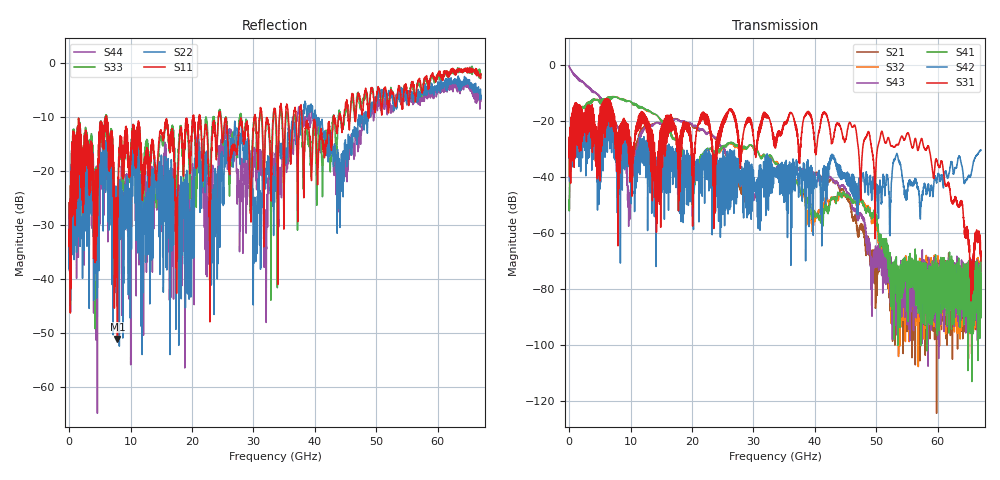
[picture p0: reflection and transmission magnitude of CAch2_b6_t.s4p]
!Agilent Technologies,N5247A,US51170199,A.09.90.13
!Agilent N5247A: A.09.90.13
!Date: Tuesday, October 23, 2018 12:56:16
!Correction: S11(Full 4 Port(1,2,3,4))
!S12(Full 4 Port(1,2,3,4))
!S13(Full 4 Port(1,2,3,4))
!S14(Full 4 Port(1,2,3,4))
!S21(Full 4 Port(1,2,3,4))
!S22(Full 4 Port(1,2,3,4))
!S23(Full 4 Port(1,2,3,4))
!S24(Full 4 Port(1,2,3,4))
!S31(Full 4 Port(1,2,3,4))
!S32(Full 4 Port(1,2,3,4))
!S33(Full 4 Port(1,2,3,4))
!S34(Full 4 Port(1,2,3,4))
!S41(Full 4 Port(1,2,3,4))
!S42(Full 4 Port(1,2,3,4))
!S43(Full 4 Port(1,2,3,4))
!S44(Full 4 Port(1,2,3,4))
!S4P File: Measurements: <S11,S12,S13,S14>,
!<S21,S22,S23,S24>,
!<S31,S32,S33,S34>,
!<S41,S42,S43,S44>:
# Hz S  dB  R 50
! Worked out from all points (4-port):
!   6701 points, 10 MHz to 67 GHz, reference 50 ohm
!   strongest paths, dB at 10 MHz, 16.76 GHz, 33.51 GHz, 50.25 GHz, 67 GHz:
!     S31: -33.0, -22.9, -27.3, -29.1, -70.0
!     S42: -33.4, -33.4, -36.8, -50.6, -30.5
!     S41: -48.3, -25.6, -35.4, -57.9, -68.5
!     S43: -0.5, -19.7, -37.8, -66.1, -68.7
!     S32: -48.4, -25.3, -35.1, -59.1, -70.9
!     S21: -0.5, -19.5, -37.4, -69.5, -80.2
!   lowest |S11| = -51.0 dB at 7.869 GHz (marker M1), VSWR 1.01, Z = 50.3 + j0.0174 ohm
!   |S11| at or under -10 dB: start of sweep to 5.977 GHz; 6.104 GHz to 20.16 GHz (14.05 GHz wide, 107 % of centre); 24.68 GHz to 30.15 GHz (5.474 GHz wide, 20 % of centre)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
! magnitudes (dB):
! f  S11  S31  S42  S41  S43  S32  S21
! 10 MHz  -25.9  -33.0  -33.4  -48.3  -0.5  -48.4  -0.5
! 7.869 GHz  -51.0  -30.2  -38.4  -11.7  -22.2  -11.6  -22.0
! 9.839 GHz  -20.3  -30.3  -34.6  -12.9  -49.5  -13.0  -34.1
! 19.61 GHz  -17.2  -25.6  -35.6  -44.0  -20.6  -41.7  -20.8
! 29.6 GHz  -29.3  -19.7  -37.5  -28.7  -46.6  -28.8  -47.7
! 55.1 GHz  -6.0  -24.3  -44.4  -72.6  -75.4  -73.4  -74.7
! 67 GHz  -2.0  -70.0  -30.5  -68.5  -68.7  -70.9  -80.2
